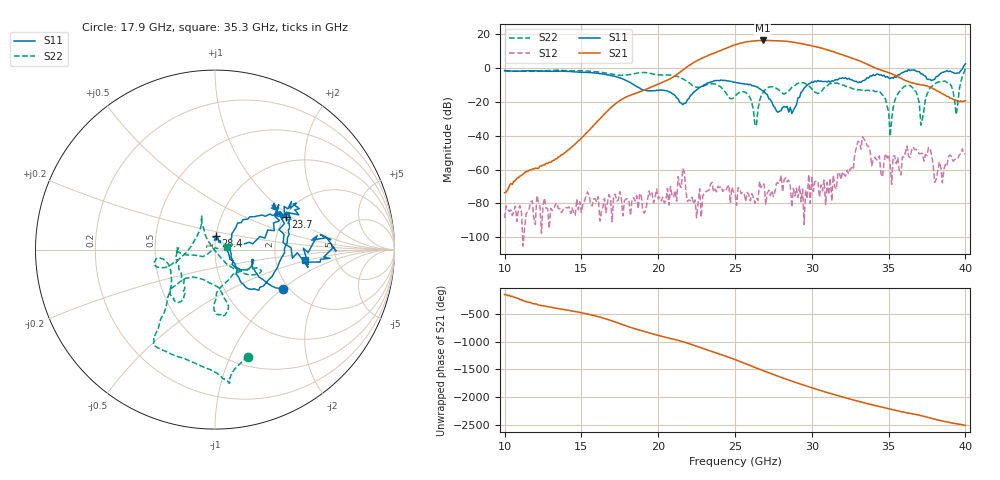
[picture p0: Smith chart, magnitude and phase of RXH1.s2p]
!Keysight Technologies,M9808A,MY58100618,A.14.70.03
!Date: Monday, February 27, 2023 13:24:16
!Correction: S11(Cdelta 2-Port  )
!S21(Cdelta 2-Port  )
!S12(Cdelta 2-Port  )
!S22(Cdelta 2-Port  )
!S2P File: Measurements: S11, S21, S12, S22:
# Hz S  RI  R 50
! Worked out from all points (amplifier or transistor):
!   301 points, 10 GHz to 40 GHz, reference 50 ohm
!   highest |S21| = 16.4 dB at 26.8 GHz (marker M1)
!   |S21| within 3 dB of that: 24.87 GHz to 29.9 GHz (5.037 GHz wide, 18.4 % of centre)
!   unconditionally stable (mu >= 1): start of sweep to 39.82 GHz
!   at 15 GHz: K = 132142.96, MAG = -32.2 dB, |S12| = -85.4 dB
!   at 25 GHz: K = 415.63, MAG = 14.7 dB, |S12| = -73.9 dB
!   at 40 GHz: K = -92.31, MSG = 15.6 dB, |S12| = -50.5 dB
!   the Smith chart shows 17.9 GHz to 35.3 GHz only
!   S11 on the Smith chart (normalised r, x): 17.9 GHz: 1.85, -1.02; 23.7 GHz: 2.03, +0.90; 28.4 GHz: 1.00, +0.15; 35.3 GHz: 2.97, -0.47
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1e10  -0.0215 0.8582  -0.00019 -8.53e-05  -3.27e-05 -1.68e-05  0.733 0.3616
1.5e10  0.7287 0.2058  -0.00467 -0.0073  2.88e-05 -4.56e-05  0.6384 -0.5504
1.79e10  0.3778 -0.2218  0.1406 0.00573  -6.71e-05 0.000117  0.1851 -0.5967
2e10  0.2091 -0.0665  -0.3334 -0.0623  -8.64e-06 0.000137  -0.129 -0.6255
2.27e10  0.1947 0.1832  1.684 -0.7309  0.000272 -2.75e-05  -0.263 -0.0763
2.37e10  0.3934 0.1798  -1.316 -2.555  -0.000225 0.000142  -0.3258 -0.0978
2.45e10  0.4086 0.1079  -3.98 0.835  0.000138 0.000266  -0.1589 -0.0156
2.5e10  0.3875 -0.0169  -2.239 4.392  -0.000173 0.000107  -0.0799 0.1234
2.55e10  0.3176 -0.1505  2.591 5.056  -0.00021 5.46e-05  -0.0741 0.1874
2.6e10  0.2433 -0.2265  6.179 0.8203  -9.63e-05 -7.06e-05  -0.0619 0.1134
2.63e10  0.1903 -0.2195  5.866 -2.76  3.61e-05 -9.37e-05  -0.0148 0.0131
2.68e10  0.1359 -0.1648  1.163 -6.537  3.89e-05 -0.000376  0.1374 -0.116
2.76e10  0.0676 -0.00607  -6.268 -1.943  -9.32e-05 -0.000196  0.2484 -0.1076
2.84e10  0.00507 0.0737  -2.876 5.543  5.03e-05 -0.000431  0.0542 -0.1884
2.93e10  0.1899 0.0409  4.509 2.938  3.21e-05 0.000109  0.0317 -0.3624
3e10  0.3602 0.1615  3.946 -2.34  5.24e-05 0.00059  0.0377 -0.2414
3.07e10  0.3331 0.2295  -0.0734 -3.868  -0.000209 -0.000104  -0.1637 -0.1599
3.15e10  0.3991 0.2096  -2.738 -1.188  5.31e-05 -0.000295  -0.2317 -0.2789
3.27e10  0.3871 0.193  -0.7027 1.8  -0.000939 -0.000376  -0.1716 -0.1709
3.5e10  0.5186 -0.0163  0.5214 -0.5276  -0.00269 -0.000777  -0.0444 -0.0273
3.53e10  0.5035 -0.0584  0.2617 -0.5943  0.00178 0.00177  0.0674 0.014
4e10  1.068 -0.8409  0.105 0.0233  -0.0019 0.00229  0.4772 -0.838
